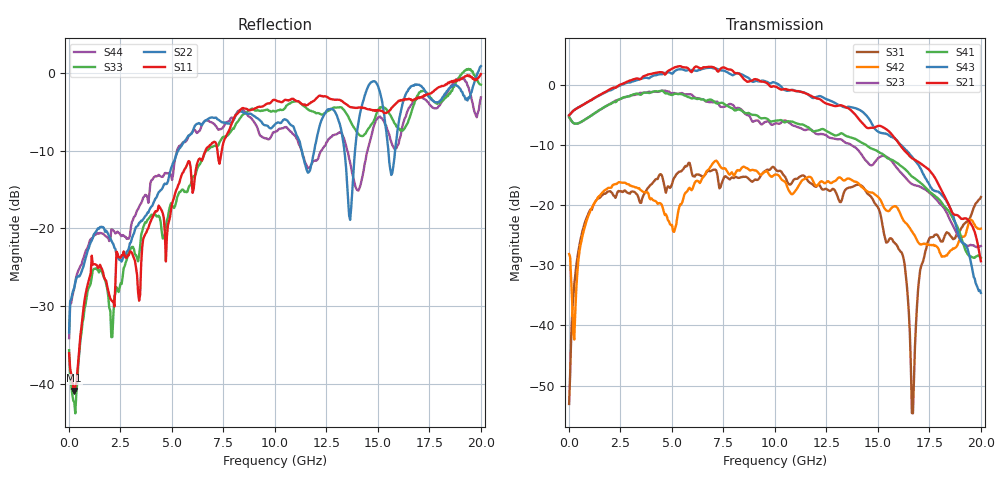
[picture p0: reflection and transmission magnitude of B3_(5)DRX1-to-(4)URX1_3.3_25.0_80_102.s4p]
!Agilent Technologies,N5225A,MY51451112,A.09.50.13
!Agilent N5225A: A.09.50.13
!Date: Sunday, March 12, 2017 05:21:46
!Correction: S11(Full 4 Port(1,2,3,4))
!S12(Full 4 Port(1,2,3,4))
!S13(Full 4 Port(1,2,3,4))
!S14(Full 4 Port(1,2,3,4))
!S21(Full 4 Port(1,2,3,4))
!S22(Full 4 Port(1,2,3,4))
!S23(Full 4 Port(1,2,3,4))
!S24(Full 4 Port(1,2,3,4))
!S31(Full 4 Port(1,2,3,4))
!S32(Full 4 Port(1,2,3,4))
!S33(Full 4 Port(1,2,3,4))
!S34(Full 4 Port(1,2,3,4))
!S41(Full 4 Port(1,2,3,4))
!S42(Full 4 Port(1,2,3,4))
!S43(Full 4 Port(1,2,3,4))
!S44(Full 4 Port(1,2,3,4))
!S4P File: Measurements: <S11,S12,S13,S14>,
!<S21,S22,S23,S24>,
!<S31,S32,S33,S34>,
!<S41,S42,S43,S44>:
# Hz S  dB  R 50
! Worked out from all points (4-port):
!   401 points, 10 MHz to 20 GHz, reference 50 ohm
!   strongest paths, dB at 10 MHz, 5.008 GHz, 10.01 GHz, 15 GHz, 20 GHz:
!     S21: -5.0, 2.7, -0.2, -6.8, -29.3
!     S43: -5.0, 1.9, 0.4, -7.7, -34.6
!     S41: -5.3, -1.7, -5.9, -11.1, -28.8
!     S23: -5.3, -1.4, -6.4, -12.2, -26.8
!     S42: -28.1, -23.3, -14.9, -18.6, -23.9
!     S31: -53.1, -16.5, -13.9, -20.3, -18.6
!   lowest |S11| = -40.8 dB at 259.9 MHz (marker M1), VSWR 1.02, Z = 50.3 - j0.873 ohm
!   |S11| at or under -10 dB: start of sweep to 6.634 GHz; 7.209 GHz to 7.421 GHz (211.2 MHz wide, 2.89 % of centre)
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1e7  -36.03 -37.9  -64.68 112.9  -52.27 16.6  -65.17 131.7
     -5.01 1.5  -33.37 39.8  -5.33 -179.9  -28.02 37.7
     -53.07 10.5  -65.37 154.6  -35.64 -45.7  -68.20 118.7
     -5.33 -179.8  -28.11 37.8  -5.00 1.6  -34.09 44.1
2.59875e8  -40.83 -72.8  -49.99 56.2  -33.16 94.9  -50.80 52.2
           -4.15 -1.2  -27.62 -131.7  -6.38 171.0  -41.86 -161.1
           -33.21 95.4  -49.74 58.2  -42.31 -79.1  -50.71 54.5
           -6.38 170.2  -42.34 -171.4  -4.14 -2.0  -27.67 -137.7
5.157425e9  -15.49 88.4  -37.78 12.0  -15.45 29.0  -39.43 -18.6
            2.98 172.3  -10.99 143.9  -1.37 -26.5  -24.25 57.8
            -15.22 27.3  -37.61 1.8  -17.09 103.8  -38.64 -54.6
            -1.45 -42.3  -23.83 59.2  2.37 162.4  -11.01 122.8
8.255875e9  -5.03 36.9  -39.72 -109.3  -15.61 -0.2  -36.37 -138.7
            1.91 19.4  -5.05 80.8  -3.83 -163.3  -13.86 47.4
            -15.45 -0.9  -32.45 -115.8  -6.07 58.6  -31.73 -151.7
            -4.04 173.6  -14.23 50.2  1.94 6.6  -4.86 45.5
1.215392e10  -2.95 -17.6  -33.38 -149.0  -16.21 -21.1  -34.63 170.7
             -2.32 -147.2  -7.01 66.8  -8.18 33.6  -16.04 40.3
             -16.58 -20.2  -34.09 -142.1  -5.22 -3.5  -33.17 175.3
             -7.50 -2.3  -16.30 43.0  -1.83 -171.3  -10.57 -6.3
1.670165e10  -3.52 -75.7  -34.80 117.9  -51.78 30.8  -36.65 86.1
             -12.28 10.8  -1.63 65.9  -16.56 167.8  -24.78 57.1
             -54.62 96.0  -33.13 121.7  -4.41 -82.3  -33.12 84.0
             -15.32 115.2  -24.62 57.1  -12.14 -38.8  -3.70 -61.2
2e10  -0.18 -114.1  -33.05 63.1  -18.65 121.3  -35.44 21.4
      -29.31 -145.9  0.84 17.1  -26.78 32.7  -23.90 101.9
      -18.63 121.3  -33.98 40.3  -1.54 -87.6  -35.27 -7.7
      -28.75 -12.1  -23.90 102.8  -34.58 -172.7  -3.17 -136.4
